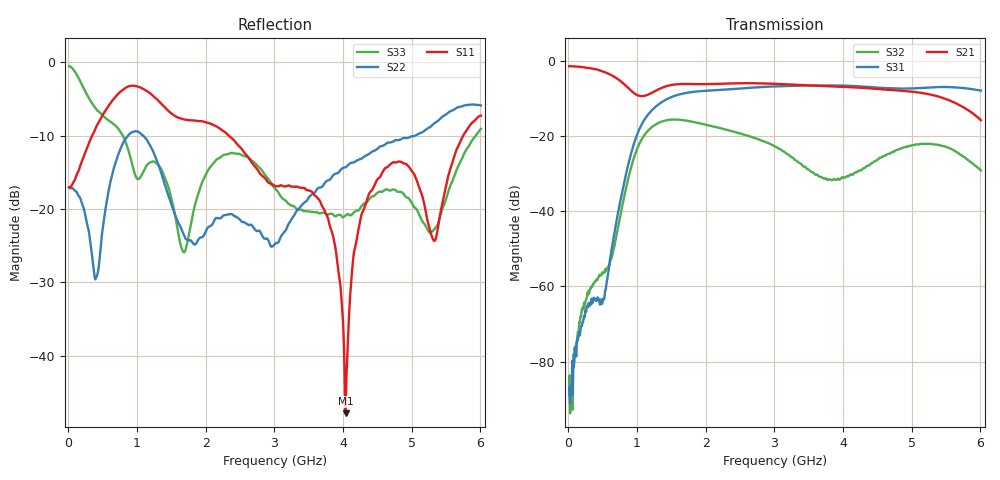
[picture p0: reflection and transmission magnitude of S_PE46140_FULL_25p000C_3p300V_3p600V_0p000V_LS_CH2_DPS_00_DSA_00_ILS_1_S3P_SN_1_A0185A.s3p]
! Device ID: PE46140_FULL
! File Path: z:\PE46140\MajorStates\25p000C\3p300\LS_CH2_DPS_00_DSA_00_ILS_1\PE46140_FULL_25p000C_3p300V_3p600V_0p000V_LS_CH2_DPS_00_DSA_00_ILS_1_S3P_SN_1_A0185A.s3p
! Serial: 1
! Lot: A0185A
! Temp: 25.000C
! VDD: 3.300
! VSS: 0.000
! Control_Hi: 3.600
! Control_Lo: 0.000
! Logic State: LS_CH2_DPS_00_DSA_00_ILS_1
! Port 1: RFIN
! Port 2: RFOUT1
! Port 3: RFOUT2
! ThroughPath:1-3
! IDD: 0.0003147198
! ISS: -1.943e-007
! Comment:
#  Hz  S  RI  R  50
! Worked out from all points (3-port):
!   801 points, 10 MHz to 6.01 GHz, reference 50 ohm
!   strongest paths, dB at 10 MHz, 1.51 GHz, 3.01 GHz, 4.51 GHz, 6.01 GHz:
!     S21: -1.5, -6.5, -6.2, -7.6, -15.9
!     S31: -86.9, -9.6, -6.8, -7.2, -8.0
!     S32: -88.9, -15.7, -22.8, -26.2, -29.2
!   lowest |S11| = -47.9 dB at 4.037 GHz (marker M1), VSWR 1.01, Z = 49.6 + j0.161 ohm
!   |S11| at or under -10 dB: start of sweep to 346.1 MHz; 2.336 GHz to 5.752 GHz (3.416 GHz wide, 84.5 % of centre)
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1e7  0.1401 -0.0108  0.842 -0.0244  -2.96e-05 4.42e-05
     0.8418 -0.0242  0.1399 -0.00678  6.78e-05 -3.92e-06
     2.45e-05 3.8e-05  3.3e-05 -1.37e-05  0.9356 -0.0889
3.55e8  -0.016 -0.3218  0.4592 -0.6283  -0.000541 -0.000247
        0.4593 -0.6263  -0.00912 -0.0426  -0.000163 0.001
        -0.000591 -0.000318  -0.000135 0.00105  -0.4605 -0.2319
1.165e9  -0.5854 0.2236  -0.205 -0.2878  -0.1915 -0.0284
         -0.2052 -0.2883  0.2134 -0.187  -0.00272 0.1186
         -0.1919 -0.0286  -0.00287 0.1185  0.1664 0.1173
1.9825e9  -0.1853 0.3454  -0.4178 0.2482  0.3911 -0.0582
          -0.4179 0.248  0.0621 -0.0261  -0.1409 -0.0173
          0.3913 -0.0581  -0.1408 -0.0174  0.0414 0.1589
3.01e9  0.0204 0.1418  0.4091 0.2722  -0.3921 -0.2291
        0.4087 0.273  -0.0577 -0.00148  0.0646 -0.0323
        -0.3924 -0.2295  0.0646 -0.0323  0.1308 -0.043
3.76e9  0.0239 0.0882  0.2811 -0.3599  -0.2495 0.3948
        0.2817 -0.3594  0.0764 0.134  -0.0161 0.0214
        -0.2495 0.3947  -0.0161 0.0215  0.0905 -0.0136
4.0375e9  -0.00371 0.00162  0.0429 -0.4428  -0.00738 0.4639
          0.0433 -0.443  0.1394 0.1324  0.024 0.0154
          -0.00635 0.4637  0.024 0.0152  0.0888 -0.0161
4.39e9  -0.1054 -0.0747  -0.258 -0.3408  0.2739 0.3519
        -0.2581 -0.3409  0.2177 0.098  0.0144 -0.0385
        0.2742 0.3515  0.0147 -0.0383  0.1139 -0.0291
5.335e9  -0.0403 -0.0452  -0.108 0.3257  0.3253 -0.3003
         -0.109 0.3258  0.383 -0.0376  0.0119 0.076
         0.3254 -0.2998  0.0118 0.0761  0.0721 0.0114
6.01e9  -0.2982 -0.3127  0.1534 0.0482  -0.1989 -0.3439
        0.1536 0.0487  0.2472 -0.4433  0.0293 -0.0188
        -0.2006 -0.3449  0.0291 -0.0189  0.3227 0.1397
